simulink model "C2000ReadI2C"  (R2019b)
settings: Solver=FixedStepDiscrete  StartTime=0.0  StopTime=Inf  RelTol=1e-3  EnableMultiTasking=on
undefined symbols (not defined in the file or in its folder): After, Before, Code, Custom, hex2dec, Write
libraries: simulink x2, c280xlib x2, idelinklib_common x1

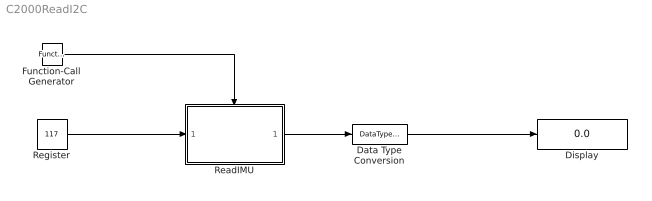
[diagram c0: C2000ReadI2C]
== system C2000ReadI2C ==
  Data Type Conversion : DataTypeConversion  OutDataTypeStr=uint16
  Display : Display
  Function-Call Generator : simulink/Ports & Subsystems/Function-Call Generator  sample_time=0.05  numberOfIterations=1
  ReadIMU : Subsystem
  Register : Constant  Value=117  OutDataTypeStr=uint16  SampleTime=-1
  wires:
  Register/1 -> ReadIMU/1(Reg)
  Function-Call Generator/1 -> ReadIMU/Trigger
  ReadIMU/1(Rx) -> Data Type Conversion/1
  Data Type Conversion/1 -> Display/1

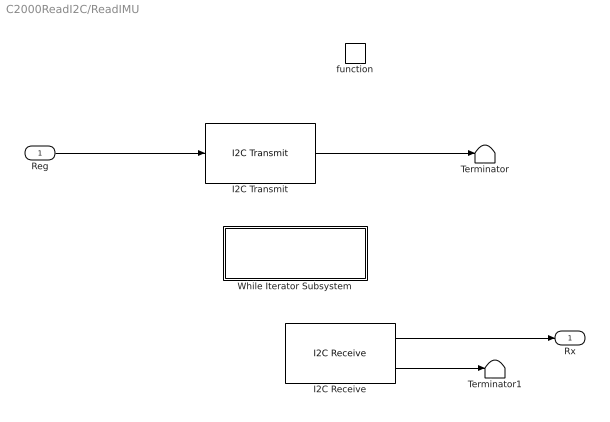
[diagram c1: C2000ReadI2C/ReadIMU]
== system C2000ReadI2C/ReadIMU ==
  Reg : Inport
  function : TriggerPort  TriggerType=function-call  VariantControl=Variant  StatesWhenEnabling=reset
  I2C Receive : c280xlib/I2C Receive  Priority=30  selectModule=I2C_A  addrFormat=7-Bit addressing  saSource=Specify via dialog  SAR=104  bitCount=8  dataLength=1  initValue=0  NACK=off  STP=on  STR=on  sampleTime=-1  dataType=uint8
  I2C Transmit : c280xlib/I2C Transmit  Priority=10  selectModule=I2C_A  addrFormat=7-Bit addressing  saSource=Specify via dialog  SAR=104  bitCount=8  STP=off  RM=off  STR=on
  Terminator : Terminator
  Terminator1 : Terminator
  While Iterator Subsystem : Subsystem  Priority=20  TreatAsAtomicUnit=on
  Rx : Outport
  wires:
  Reg/1 -> I2C Transmit/1
  I2C Receive/1 -> Rx/1
  I2C Transmit/1 -> Terminator/1
  I2C Receive/2 -> Terminator1/1

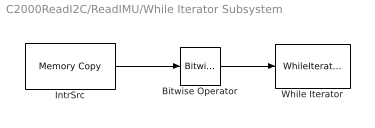
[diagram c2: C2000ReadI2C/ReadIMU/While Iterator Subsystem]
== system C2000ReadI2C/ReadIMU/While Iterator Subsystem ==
  Bitwise Operator : simulink/Logic and Bit Operations/Bitwise Operator  logicop=AND  UseBitMask=on  BitMask=hex2dec('1F00')  BitMaskRealWorld=Stored Integer
  IntrSrc : idelinklib_common/Memory Copy  copyFrom=Specified source code symbol  copyFromAddressSource=Specify via dialog  copyFromAddress=hex2dec('00001000')  copyFromSrcCode=&I2caRegs.I2CFFTX.all  dataTypeFrom=uint16  dataDimensionFrom=1  useOffsetFrom=off  offsetFromSrc=Specify via dialog  offsetFrom=1  strideFrom=1  copyTo=Output port  copyToAddressSource=Specify via dialog  copyToAddress=hex2dec('00002000')  copyToSrcCode=myVariableDst  dataTypeTo=uint16  useOffsetTo=off  offsetToSrc=Specify via dialog  offsetTo=1  strideTo=1  sampleTime=-1  useInitValue=off  initValueSrc=Specify constant value  initValue=1  initValueSrcCode=myInitValueVariable  useAsMask=off  maskOperator=bitwise AND  useTermValue=off  termValue=1  isRealtimeEnabled=off  emitCCBeforeWrite=off  CCBeforeWrite=/* Custom Code Before Write*/  emitCCAfterWrite=off  CCAfterWrite=/* Custom Code After Write*/  useDMACopy=off  enableBlockingMode=off
  While Iterator : WhileIterator  MaxIters=-1  WhileBlockType=do-while
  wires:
  IntrSrc/1 -> Bitwise Operator/1
  Bitwise Operator/1 -> While Iterator/1
